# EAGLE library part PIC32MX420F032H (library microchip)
PIC32MX420F032H edit this description Auto generated by make-symbol-device-package-bsdl.ulp Rev. 25 Source: PIC32MX420F032H.bsdl
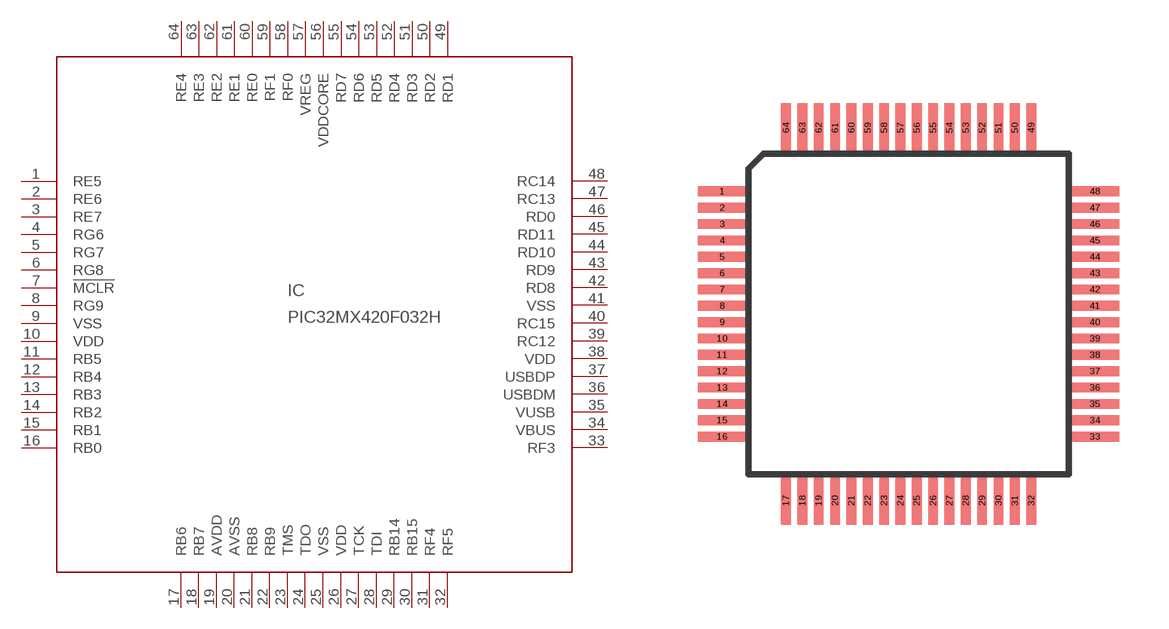
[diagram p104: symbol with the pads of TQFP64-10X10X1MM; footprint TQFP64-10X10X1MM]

Designator prefix IC

## PIC32MX420F032H (MF: MICROCHIP; MPN: PIC32MX420F032H-40I/PT; OC_FARNELL: 1640230; OC_NEWARK: 98M1932)  [TQFP64-10X10X1MM]
1  RE5
2  RE6
3  RE7
4  RG6
5  RG7
6  RG8
7  !MCLR  in
8  RG9
9  VSS  pwr
10  VDD  pwr
11  RB5
12  RB4
13  RB3
14  RB2
15  RB1
16  RB0
17  RB6
18  RB7
19  AVDD  pwr
20  AVSS  pwr
21  RB8
22  RB9
23  TMS  in
24  TDO  out
25  VSS  pwr
26  VDD  pwr
27  TCK  in
28  TDI  in
29  RB14
30  RB15
31  RF4
32  RF5
33  RF3
34  VBUS
35  VUSB  pas
36  USBDM
37  USBDP
38  VDD  pwr
39  RC12
40  RC15
41  VSS  pwr
42  RD8
43  RD9
44  RD10
45  RD11
46  RD0
47  RC13
48  RC14
49  RD1
50  RD2
51  RD3
52  RD4
53  RD5
54  RD6
55  RD7
56  VDDCORE  pwr
57  VREG  pas
58  RF0
59  RF1
60  RE0
61  RE1
62  RE2
63  RE3
64  RE4

## Footprint TQFP64-10X10X1MM (pad centres in mm)
64-Lead Plastic Thin Quad Flatpak (PT) - 10x10x1 mm Body Auto generated by make-symbol-device-package-bsdl.ulp Rev. 37 Source: http://ww1.microchip.com/downloads/en/DeviceDoc/61143G.pdf
smd 1.5 x 0.3: 1 -5.7,3.75; 2 -5.7,3.25; 3 -5.7,2.75; 4 -5.7,2.25; 5 -5.7,1.75; 6 -5.7,1.25; 7 -5.7,0.75; 8 -5.7,0.25; 9 -5.7,-0.25; 10 -5.7,-0.75; 11 -5.7,-1.25; 12 -5.7,-1.75; 13 -5.7,-2.25; 14 -5.7,-2.75; 15 -5.7,-3.25; 16 -5.7,-3.75; 33 5.7,-3.75; 34 5.7,-3.25; 35 5.7,-2.75; 36 5.7,-2.25; 37 5.7,-1.75; 38 5.7,-1.25; 39 5.7,-0.75; 40 5.7,-0.25; 41 5.7,0.25; 42 5.7,0.75; 43 5.7,1.25; 44 5.7,1.75; 45 5.7,2.25; 46 5.7,2.75; 47 5.7,3.25; 48 5.7,3.75
smd 0.3 x 1.5: 17 -3.75,-5.7; 18 -3.25,-5.7; 19 -2.75,-5.7; 20 -2.25,-5.7; 21 -1.75,-5.7; 22 -1.25,-5.7; 23 -0.75,-5.7; 24 -0.25,-5.7; 25 0.25,-5.7; 26 0.75,-5.7; 27 1.25,-5.7; 28 1.75,-5.7; 29 2.25,-5.7; 30 2.75,-5.7; 31 3.25,-5.7; 32 3.75,-5.7; 49 3.75,5.7; 50 3.25,5.7; 51 2.75,5.7; 52 2.25,5.7; 53 1.75,5.7; 54 1.25,5.7; 55 0.75,5.7; 56 0.25,5.7; 57 -0.25,5.7; 58 -0.75,5.7; 59 -1.25,5.7; 60 -1.75,5.7; 61 -2.25,5.7; 62 -2.75,5.7; 63 -3.25,5.7; 64 -3.75,5.7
